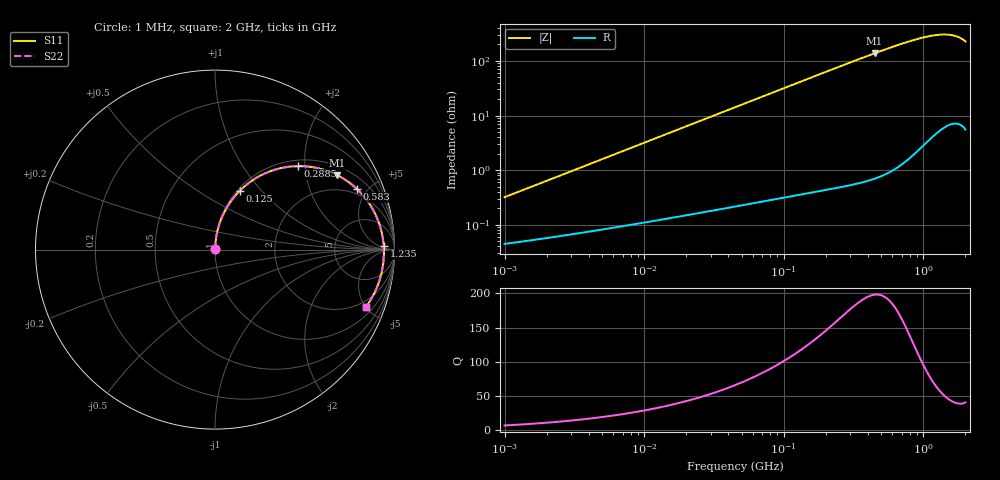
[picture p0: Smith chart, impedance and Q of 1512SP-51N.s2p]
# MHz  S  MA  R  50
!Freq  MagS11  AngS11  MagS21  AngS21  MagS12  AngS12  MagS22  AngS22
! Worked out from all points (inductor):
!   801 points, 1 MHz to 2 GHz, reference 50 ohm
!   read as one part in series: L = 50.4 nH near 1.039 MHz
!   highest Q = 198 at 446.8 MHz (marker M1), where L = 49 nH
!   S11 on the Smith chart (normalised r, x): 1 MHz: 1.00, +0.01; 125 MHz: 1.03, +0.77; 288.5 MHz: 1.13, +1.84; 583 MHz: 1.65, +4.28; 1.235 GHz: 29, +10; 2 GHz: 1.51, -5.05
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1  0.003094 81.5  0.9996 -0.2  0.9996 -0.2  0.003094 81.5
3.573795  0.01096 85.6  0.9992 -0.7  0.9992 -0.7  0.01096 85.6
12.65119  0.0387 85.8  0.998 -2.4  0.998 -2.4  0.03869 85.8
25.31997  0.07722 84.0  0.9954 -4.7  0.9954 -4.7  0.0772 84.0
44.78507  0.1356 80.8  0.9886 -8.3  0.9886 -8.3  0.1356 80.8
79.97073  0.2372 74.7  0.9688 -14.7  0.9688 -14.7  0.2371 74.7
125.0084  0.3559 67.1  0.9313 -22.3  0.9313 -22.3  0.3558 67.1
160.0527  0.4377 61.7  0.8957 -27.9  0.8957 -27.9  0.4375 61.7
221.1104  0.5566 53.1  0.8271 -36.5  0.8271 -36.5  0.5563 53.1
288.5284  0.6563 45.2  0.7508 -44.5  0.7508 -44.5  0.6558 45.2
359.0283  0.7321 38.3  0.6774 -51.4  0.6774 -51.4  0.7316 38.3
446.7544  0.7978 31.3  0.5992 -58.4  0.5992 -58.4  0.7971 31.3
566.5845  0.8545 24.0  0.5153 -65.7  0.5153 -65.7  0.8538 24.0
582.9727  0.8603 23.1  0.5056 -66.6  0.5056 -66.6  0.8595 23.1
698.3562  0.8917 17.8  0.4477 -71.9  0.4477 -71.9  0.8908 17.8
844.5662  0.9159 12.3  0.3948 -77.3  0.3948 -77.3  0.9149 12.3
1021.387  0.932 6.8  0.3527 -82.5  0.3527 -82.5  0.9309 6.8
1235.228  0.9405 1.1  0.3248 -87.9  0.3248 -87.9  0.9393 1.1
1424.507  0.9413 -3.6  0.3171 -92.4  0.3171 -92.4  0.9402 -3.6
1611.856  0.9367 -8.4  0.3243 -96.9  0.3243 -96.9  0.9357 -8.4
1789.503  0.9261 -13.4  0.347 -101.7  0.347 -101.7  0.9252 -13.4
2000  0.9002 -20.7  0.4012 -109.0  0.4012 -109.0  0.8996 -20.7
